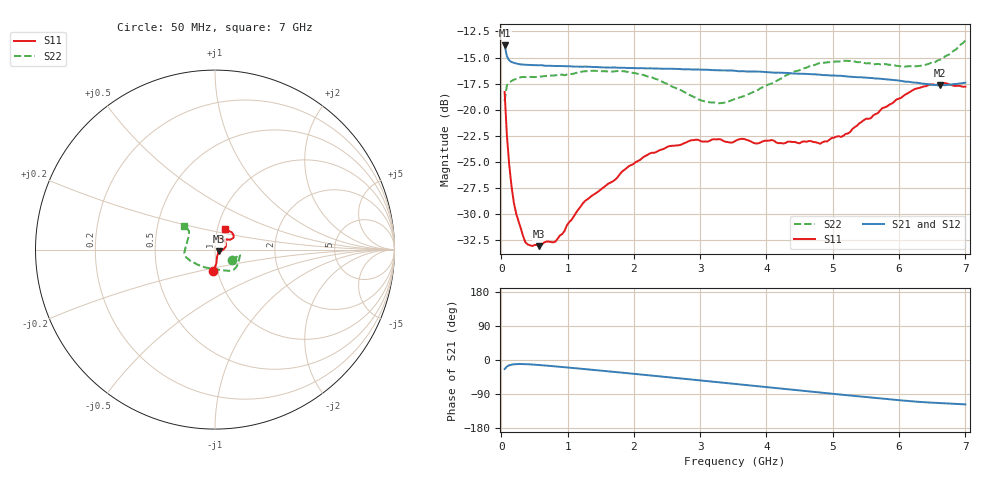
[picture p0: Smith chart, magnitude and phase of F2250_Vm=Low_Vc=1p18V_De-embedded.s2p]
! Integrated Device Technology
! Corporate Headquarters
! 6024 Silver Creek Valley Road
! San Jose, CA 95138  USA
! Phone:  1-408-284-8200
! Toll Free:  1-800-223-1366
! Webpage:  http://www.idt.com/
! Timing and RF Division
! 515 Groton Road, Suite 102
! Westford, MA 01886-6024
! Device:  F2250
! Description: Voltage Variable RF Attenuator
! Frequency:  50.0 -  6000.00 MHz
! Package:  3x3 mm Thin QFN Plastic Package: 16 pin
! Ports:  2 RF, 3 DC
!  Pin  1  = GND
!  Pin  2  = NC
!  Pin  3  = RF1  = Port 1
!  Pin  4  = NC
!  Pin  5  = GND
!  Pin  6  = GND
!  Pin  7  = GND
!  Pin  8  = GND
!  Pin  9  = NC
!  Pin 10  = RF2  = Port 2
!  Pin 11  = NC
!  Pin 12  = GND
!  Pin 13  = GND
!  Pin 14  = VCNTRL
!  Pin 15  = VDD
!  Pin 16  = VMODE
! Vcntrl:  1.180 Volts
! Vmode:  +0.000 Volts
! Vdd:  +3.30  Volts
! Current:  1.195 mA
! Data:  The device was measured on a the F2250 evaluation board which has
!  individual transmission lines to the RF pins.  Data was collected
!  using a calibrated network analyzer.  The evaluation board was
!  de-embedded using a TRL calibration technique.
!  The reference plane is the edge of the package pin.
! Misc:  SN 10
!  Action Tracker AT0258
! Date Measured:  2014-11-26
! Date:  2015-10-15  MJV
! Note:
!  Integrated Device Technology supplies this data as a sample of measured
!  data at the package pin for this product.  Your particular data for this
!  product may vary.
!  Data was taken at 25 degrees C.
!  Integrated Device Technology reserves the right to change this data at anytime.
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# GHz S dB R 50
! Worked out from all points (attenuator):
!   201 points, 50 MHz to 7 GHz, reference 50 ohm
!   highest |S21| = -13.82 dB at 50 MHz (marker M1); lowest = -17.7 dB at 6.618 GHz (marker M2)
!   lowest |S11| = -33.1 dB at 571.2 MHz (marker M3), VSWR 1.05, Z = 52 - j1.02 ohm
!   |S11| at or under -10 dB: start of sweep to end of sweep
!   |S22| runs from -19.4 to -13.4 dB; largest |S21 - S12| = 0.00063
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0.05  -18.30 -94.2  -13.82 -23.9  -13.79 -23.9  -19.17 -32.7
0.08475  -22.49 -83.9  -14.89 -17.3  -14.88 -17.3  -17.65 -16.6
0.1195  -25.27 -79.3  -15.27 -14.0  -15.25 -14.0  -17.38 -12.4
0.15425  -27.35 -75.0  -15.43 -12.2  -15.41 -12.2  -17.26 -11.4
0.22375  -29.93 -62.2  -15.57 -10.8  -15.58 -10.8  -17.06 -11.7
0.36275  -32.69 -44.5  -15.69 -10.9  -15.70 -10.9  -16.88 -13.2
0.57125  -33.07 -26.1  -15.74 -13.2  -15.74 -13.2  -16.84 -18.6
0.8145  -32.65 -18.4  -15.82 -16.8  -15.79 -16.8  -16.71 -25.6
1.2315  -28.96 -10.9  -15.88 -23.5  -15.88 -23.5  -16.34 -35.9
1.9265  -25.39 7.3  -16.01 -35.2  -15.99 -35.2  -16.41 -48.9
2.37825  -23.91 18.7  -16.07 -42.9  -16.06 -42.9  -17.15 -58.6
2.86475  -22.93 34.3  -16.14 -51.5  -16.15 -51.5  -18.66 -76.5
3.0385  -23.06 40.7  -16.16 -54.5  -16.15 -54.5  -19.16 -85.8
3.28175  -22.82 48.5  -16.23 -58.8  -16.21 -58.8  -19.38 -101.3
3.525  -23.01 55.8  -16.28 -63.1  -16.29 -63.1  -18.97 -116.7
4.7065  -23.10 64.7  -16.61 -84.0  -16.60 -84.0  -15.75 -163.2
4.81075  -23.26 61.0  -16.65 -85.8  -16.64 -85.8  -15.53 -165.1
5.1235  -22.61 51.2  -16.75 -91.4  -16.76 -91.4  -15.37 -171.9
5.85325  -19.51 32.7  -17.12 -103.7  -17.11 -103.8  -15.70 171.9
6.2355  -18.03 33.8  -17.40 -109.5  -17.40 -109.6  -15.85 159.2
6.61775  -17.53 42.9  -17.67 -113.5  -17.66 -113.5  -15.21 146.4
7  -17.78 63.6  -17.41 -117.1  -17.42 -117.2  -13.37 142.6
